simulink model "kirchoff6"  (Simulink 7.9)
settings: Solver=ode23s  StartTime=0.0  StopTime=10  RelTol=1e-3
libraries: fl_lib x5, nesl_utility x3, powerlib x1

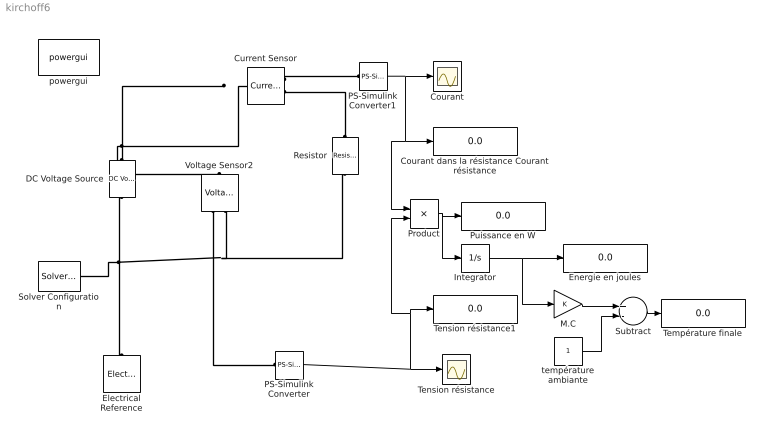
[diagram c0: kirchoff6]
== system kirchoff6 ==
  Courant : Scope
  Courant dans la résistance Courant résistance : Display
  Current Sensor : fl_lib/Electrical/Electrical Sensors/Current Sensor  i1_Log=off  v1_Log=off  LocalVarNames=|i1|v1  LocalVarDescs=|i1|v1  LocalVarLogging=[0 0]
  DC Voltage Source : fl_lib/Electrical/Electrical Sources/DC Voltage Source  v0=1 V  i_Log=off  v_Log=off  LocalVarNames=|i|v  LocalVarDescs=|i|v  LocalVarLogging=[0 0]
  Electrical Reference : fl_lib/Electrical/Electrical Elements/Electrical Reference  i_Log=off  LocalVarNames=|i  LocalVarDescs=|i  LocalVarLogging=0
  Energie en joules : Display
  Integrator : Integrator
  M.C : Gain
  PS-Simulink Converter : nesl_utility/PS-Simulink Converter  PhysicalDomain=network_engine_domain  LeftPortType=input  RightPortType=output  SubClassName=ps_output  Unit=V  AffineConversion=off
  PS-Simulink Converter1 : nesl_utility/PS-Simulink Converter  PhysicalDomain=network_engine_domain  LeftPortType=input  RightPortType=output  SubClassName=ps_output  Unit=A  AffineConversion=off
  Product : Product
  Puissance en W : Display
  Resistor : fl_lib/Electrical/Electrical Elements/Resistor  R=183 Ohm  i_Log=off  v_Log=off  LocalVarNames=|i|v  LocalVarDescs=|i|v  LocalVarLogging=[0 0]
  Solver Configuration : nesl_utility/Solver Configuration  PhysicalDomain=network_engine_domain  LeftPortType=input  RightPortType=generic  SubClassName=solver  UseCustomDae=off  DoDC=off  ResidualTolerance=1e-9  UseLocalSolver=off  LocalSolverChoice=NE_BACKWARD_EULER_ADVANCER  LocalSolverSampleTime=.001  DoFixedCost=off  MaxNonlinIter=3  MaxModeIter=2  LinearAlgebra=Sparse  Accelerate=off  Profile=off  UseLocalSampling=off  DelaysMemoryBudget=1024
  Subtract : Sum  Inputs=+-
  Température finale : Display
  Tension résistance : Scope
  Tension résistance1 : Display
  Voltage Sensor2 : fl_lib/Electrical/Electrical Sensors/Voltage Sensor  i1_Log=off  v1_Log=off  LocalVarNames=|i1|v1  LocalVarDescs=|i1|v1  LocalVarLogging=[0 0]
  powergui : powerlib/powergui  Priority=1  SimulationMode=Continuous  SolverType=Tustin  SampleTime=50e-6  frequency=60  SPID=off  DisableSnubberDevices=off  DisableRonSwitches=off  DisableVfSwitches=off  SwTol=0  Interpol=off  DisplayEquations=off  FunctionMessages=off  frequencyindice=17  Pbase=100e6  ErrMax=1e-4  Iterations=50  UnitsV=V  UnitsW=W  echomessages=off  HookPort=off  EnableUseOfTLC=off  x0status=blocks  RestoreLinks=warning  ResistiveCurrentMeasurement=off  Ylog=off  Xlog=on  ShowGrid=off  save=off  variable=ZData  ZoomFFT=off  StartTime=0.0  cycles=1  DisplayStyle=1  FreqAxis=off  MaxFrequency=1000  frequencyindicesteady=1  display=off  methode=off
  température ambiante : Constant
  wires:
  PS-Simulink Converter1/1 -> Courant/1, Courant dans la résistance Courant résistance/1, Product/1
  PS-Simulink Converter/1 -> Tension résistance/1, Tension résistance1/1, Product/2
  Product/1 -> Puissance en W/1, Integrator/1
  Integrator/1 -> Energie en joules/1, M.C/1
  M.C/1 -> Subtract/1
  température ambiante/1 -> Subtract/2
  Subtract/1 -> Température finale/1
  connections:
  Voltage Sensor2/RConn2 -- Solver Configuration/RConn1 -- Electrical Reference/LConn1 -- DC Voltage Source/RConn1 -- Resistor/RConn1
  DC Voltage Source/LConn1 -- Voltage Sensor2/LConn1 -- Current Sensor/LConn1
  Current Sensor/RConn1 -- PS-Simulink Converter1/LConn1
  Resistor/LConn1 -- Current Sensor/RConn2
  Voltage Sensor2/RConn1 -- PS-Simulink Converter/LConn1
